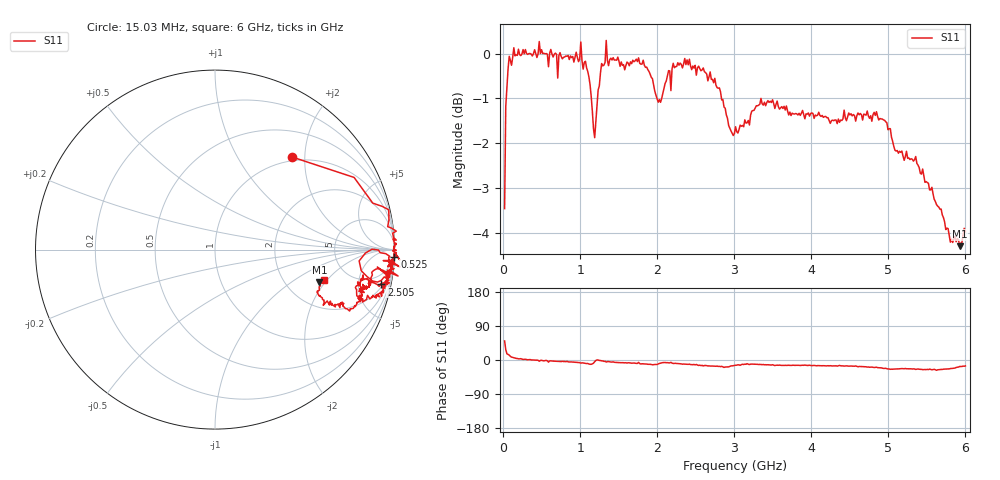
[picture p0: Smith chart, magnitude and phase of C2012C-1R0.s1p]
!	Network	Analyzer	HP8753E.07.74:	Oct	30	2002	Serial	No.	JP38451487
!	Hewlett-Packard
!	28	Aug	2009	12:15:49
!	Frequency	S11
#	HZ	S	RI	R	50
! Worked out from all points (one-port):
!   400 points, 15.03 MHz to 6 GHz, reference 50 ohm
!   lowest |S11| = -4.3 dB at 5.925 GHz (marker M1), VSWR 4.12, Z = 152 - j86.9 ohm
!   |S11| at or under -10 dB: nowhere
!   S11 on the Smith chart (normalised r, x): 15.03 MHz: 0.93, +1.74; 525 MHz: -1, -49; 2.505 GHz: 2.43, -9.00; 6 GHz: 3.30, -1.87
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1.502992e7  0.429 0.516
3.002985e7  0.775 0.402
4.502978e7  0.879 0.259
7.502962e7  0.968 0.222
1.95029e8  1.01 0.0532
5.250274e8  1 -0.0405
7.650262e8  0.985 -0.0566
1.005025e9  1.02 -0.147
1.140024e9  0.878 -0.175
1.185024e9  0.803 -0.0632
1.215024e9  0.875 0.00226
1.335023e9  1.03 -0.0961
1.515022e9  0.961 -0.115
1.755021e9  0.983 -0.11
1.785021e9  0.957 -0.177
2.01002e9  0.868 -0.159
2.175019e9  0.904 -0.0974
2.265019e9  0.964 -0.158
2.505017e9  0.926 -0.194
2.865016e9  0.821 -0.292
3.015015e9  0.804 -0.2
3.765011e9  0.832 -0.203
4.515007e9  0.824 -0.234
5.025005e9  0.75 -0.342
5.265004e9  0.702 -0.303
5.625002e9  0.603 -0.31
5.925e9  0.582 -0.18
6e9  0.609 -0.17
